(* Logix 5000 AddOnInstructionDefinition export Bronkhorst_Extended_REAL_Input; software revision 37.00 *)

ADD_ON_INSTRUCTION Bronkhorst_Extended_REAL_Input   (* revision 1.0, vendor Bronkhorst High-Tech B.V. *)
// Extract data from the Extended REAL input connection (in to controller from device)
VAR_IN_OUT
   DataIn : SINT[14]; {required}
END_VAR
VAR_OUTPUT
   Status : SINT; {visible}
   Measure : REAL; {visible}
END_VAR
VAR_INPUT
   Setpoint : REAL; {visible}
   Override : USINT; {visible}
   Actuator : REAL; {visible}
END_VAR

ROUTINE Logic   (* structured text *)
   Status := DataIn[0];
   COP(DataIn[1], Measure, 1);
   COP(DataIn[5], Setpoint, 1);
   Override := DataIn[9];
   COP(DataIn[10], Actuator, 1);
END_ROUTINE
END_ADD_ON_INSTRUCTION

ADD_ON_INSTRUCTION Bronkhorst_Extended_REAL_Output   (* revision 1.0, vendor Bronkhorst High-Tech B.V. *)
// Fill data for the Extended REAL output connection (out from controller to device)
VAR_IN_OUT
   DataOut : SINT[5]; {required}
END_VAR
VAR_INPUT
   Override : USINT; {visible}
   Setpoint : REAL; {visible}
END_VAR

ROUTINE Logic   (* structured text *)
   DataOut[0] := Override;
   COP(Setpoint, DataOut[1], 4);
END_ROUTINE
END_ADD_ON_INSTRUCTION
